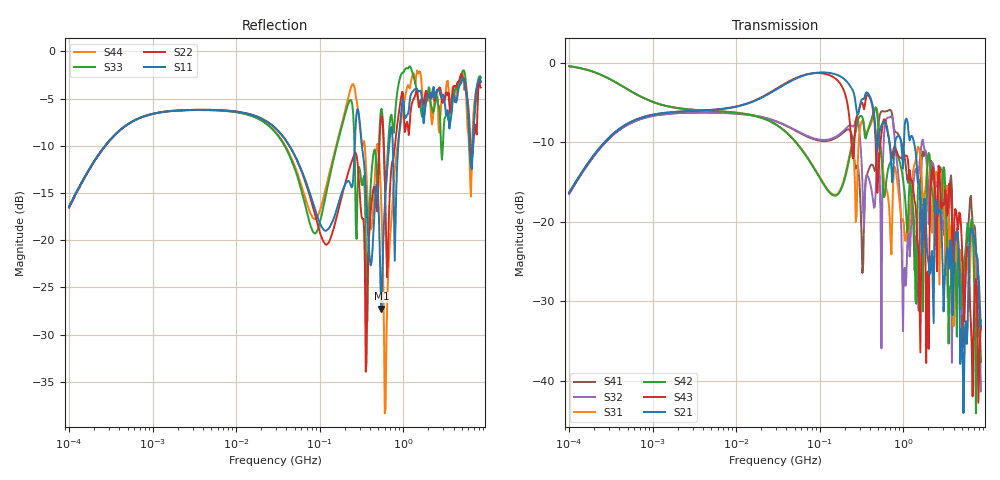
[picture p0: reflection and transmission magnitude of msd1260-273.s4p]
# MHz S MA R 50
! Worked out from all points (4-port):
!   498 points, 100 kHz to 8.5 GHz, reference 50 ohm
!   strongest paths, dB at 100 kHz, 1.698 MHz, 29.49 MHz, 500.7 MHz, 8.5 GHz:
!     S21: -16.3, -6.2, -3.4, -10.3, -32.4
!     S43: -16.3, -6.2, -3.3, -14.6, -33.1
!     S42: -0.4, -5.6, -7.7, -7.6, -37.7
!     S31: -0.4, -5.6, -7.7, -7.2, -37.1
!     S32: -16.5, -6.4, -7.3, -11.3, -41.3
!     S41: -16.5, -6.4, -7.3, -8.3, -33.5
!   lowest |S11| = -27.3 dB at 548.6 MHz (marker M1), VSWR 1.09, Z = 54.1 - j1.98 ohm
!   |S11| at or under -10 dB: 43.49 MHz to 262.6 MHz (219.1 MHz wide, 143 % of centre); 320.4 MHz to 677.7 MHz (357.3 MHz wide, 71.6 % of centre); 6.263 GHz to 6.839 GHz (575.9 MHz wide, 8.79 % of centre)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
0.1  0.1496 71.3  0.1527 70.9  0.9556 -8.7  0.1502 -109.4
     0.1527 70.9  0.1489 70.9  0.1503 -109.5  0.9563 -8.7
     0.9556 -8.7  0.1503 -109.5  0.1506 70.9  0.1526 70.8
     0.1502 -109.4  0.9563 -8.7  0.1526 70.8  0.1492 70.7
230.3138  0.201 -5.9  0.7204 -57.6  0.2725 101.6  0.3773 -7.0
          0.7204 -57.6  0.2449 -7.2  0.4052 0.2  0.262 121.3
          0.2725 101.6  0.4052 0.2  0.5505 -30.9  0.413 -80.7
          0.3773 -7.0  0.262 121.3  0.413 -80.7  0.6166 -16.0
363.6528  0.1503 -87.1  0.6544 -69.9  0.3594 12.1  0.194 18.6
          0.6544 -69.9  0.02249 38.5  0.1965 -33.3  0.3498 16.9
          0.3594 12.1  0.1965 -33.3  0.03879 -74.3  0.6219 -64.4
          0.194 18.6  0.3498 16.9  0.6219 -64.4  0.2121 -102.2
548.5512  0.04337 -25.0  0.404 -86.1  0.2634 -102.3  0.4962 -19.3
          0.404 -86.1  0.4552 -28.8  0.01596 56.8  0.255 -83.5
          0.2634 -102.3  0.01596 56.8  0.496 -27.3  0.3571 -71.4
          0.4962 -19.3  0.255 -83.5  0.3571 -71.4  0.147 -144.6
1336.696  0.621 -123.8  0.3209 166.1  0.2201 -73.8  0.07711 163.7
          0.3209 166.1  0.5612 -120.4  0.1823 -83.2  0.1082 177.0
          0.2201 -73.8  0.1823 -83.2  0.7311 -148.3  0.1514 159.9
          0.07711 163.7  0.1082 177.0  0.1514 159.9  0.7614 -122.7
3111.8  0.5476 53.7  0.03912 91.8  0.1355 -7.6  0.08201 25.4
        0.03912 91.8  0.5426 74.9  0.1242 48.0  0.2124 1.0
        0.1355 -7.6  0.1242 48.0  0.4388 75.3  0.1327 39.5
        0.08201 25.4  0.2124 1.0  0.1327 39.5  0.5768 75.5
8500  0.6893 -53.6  0.02403 -95.8  0.01394 -63.8  0.02117 -133.0
      0.02403 -95.8  0.6434 -38.8  0.008564 170.2  0.01308 -113.2
      0.01394 -63.8  0.008564 170.2  0.726 -50.6  0.02216 -17.7
      0.02117 -133.0  0.01308 -113.2  0.02216 -17.7  0.6858 -47.8
